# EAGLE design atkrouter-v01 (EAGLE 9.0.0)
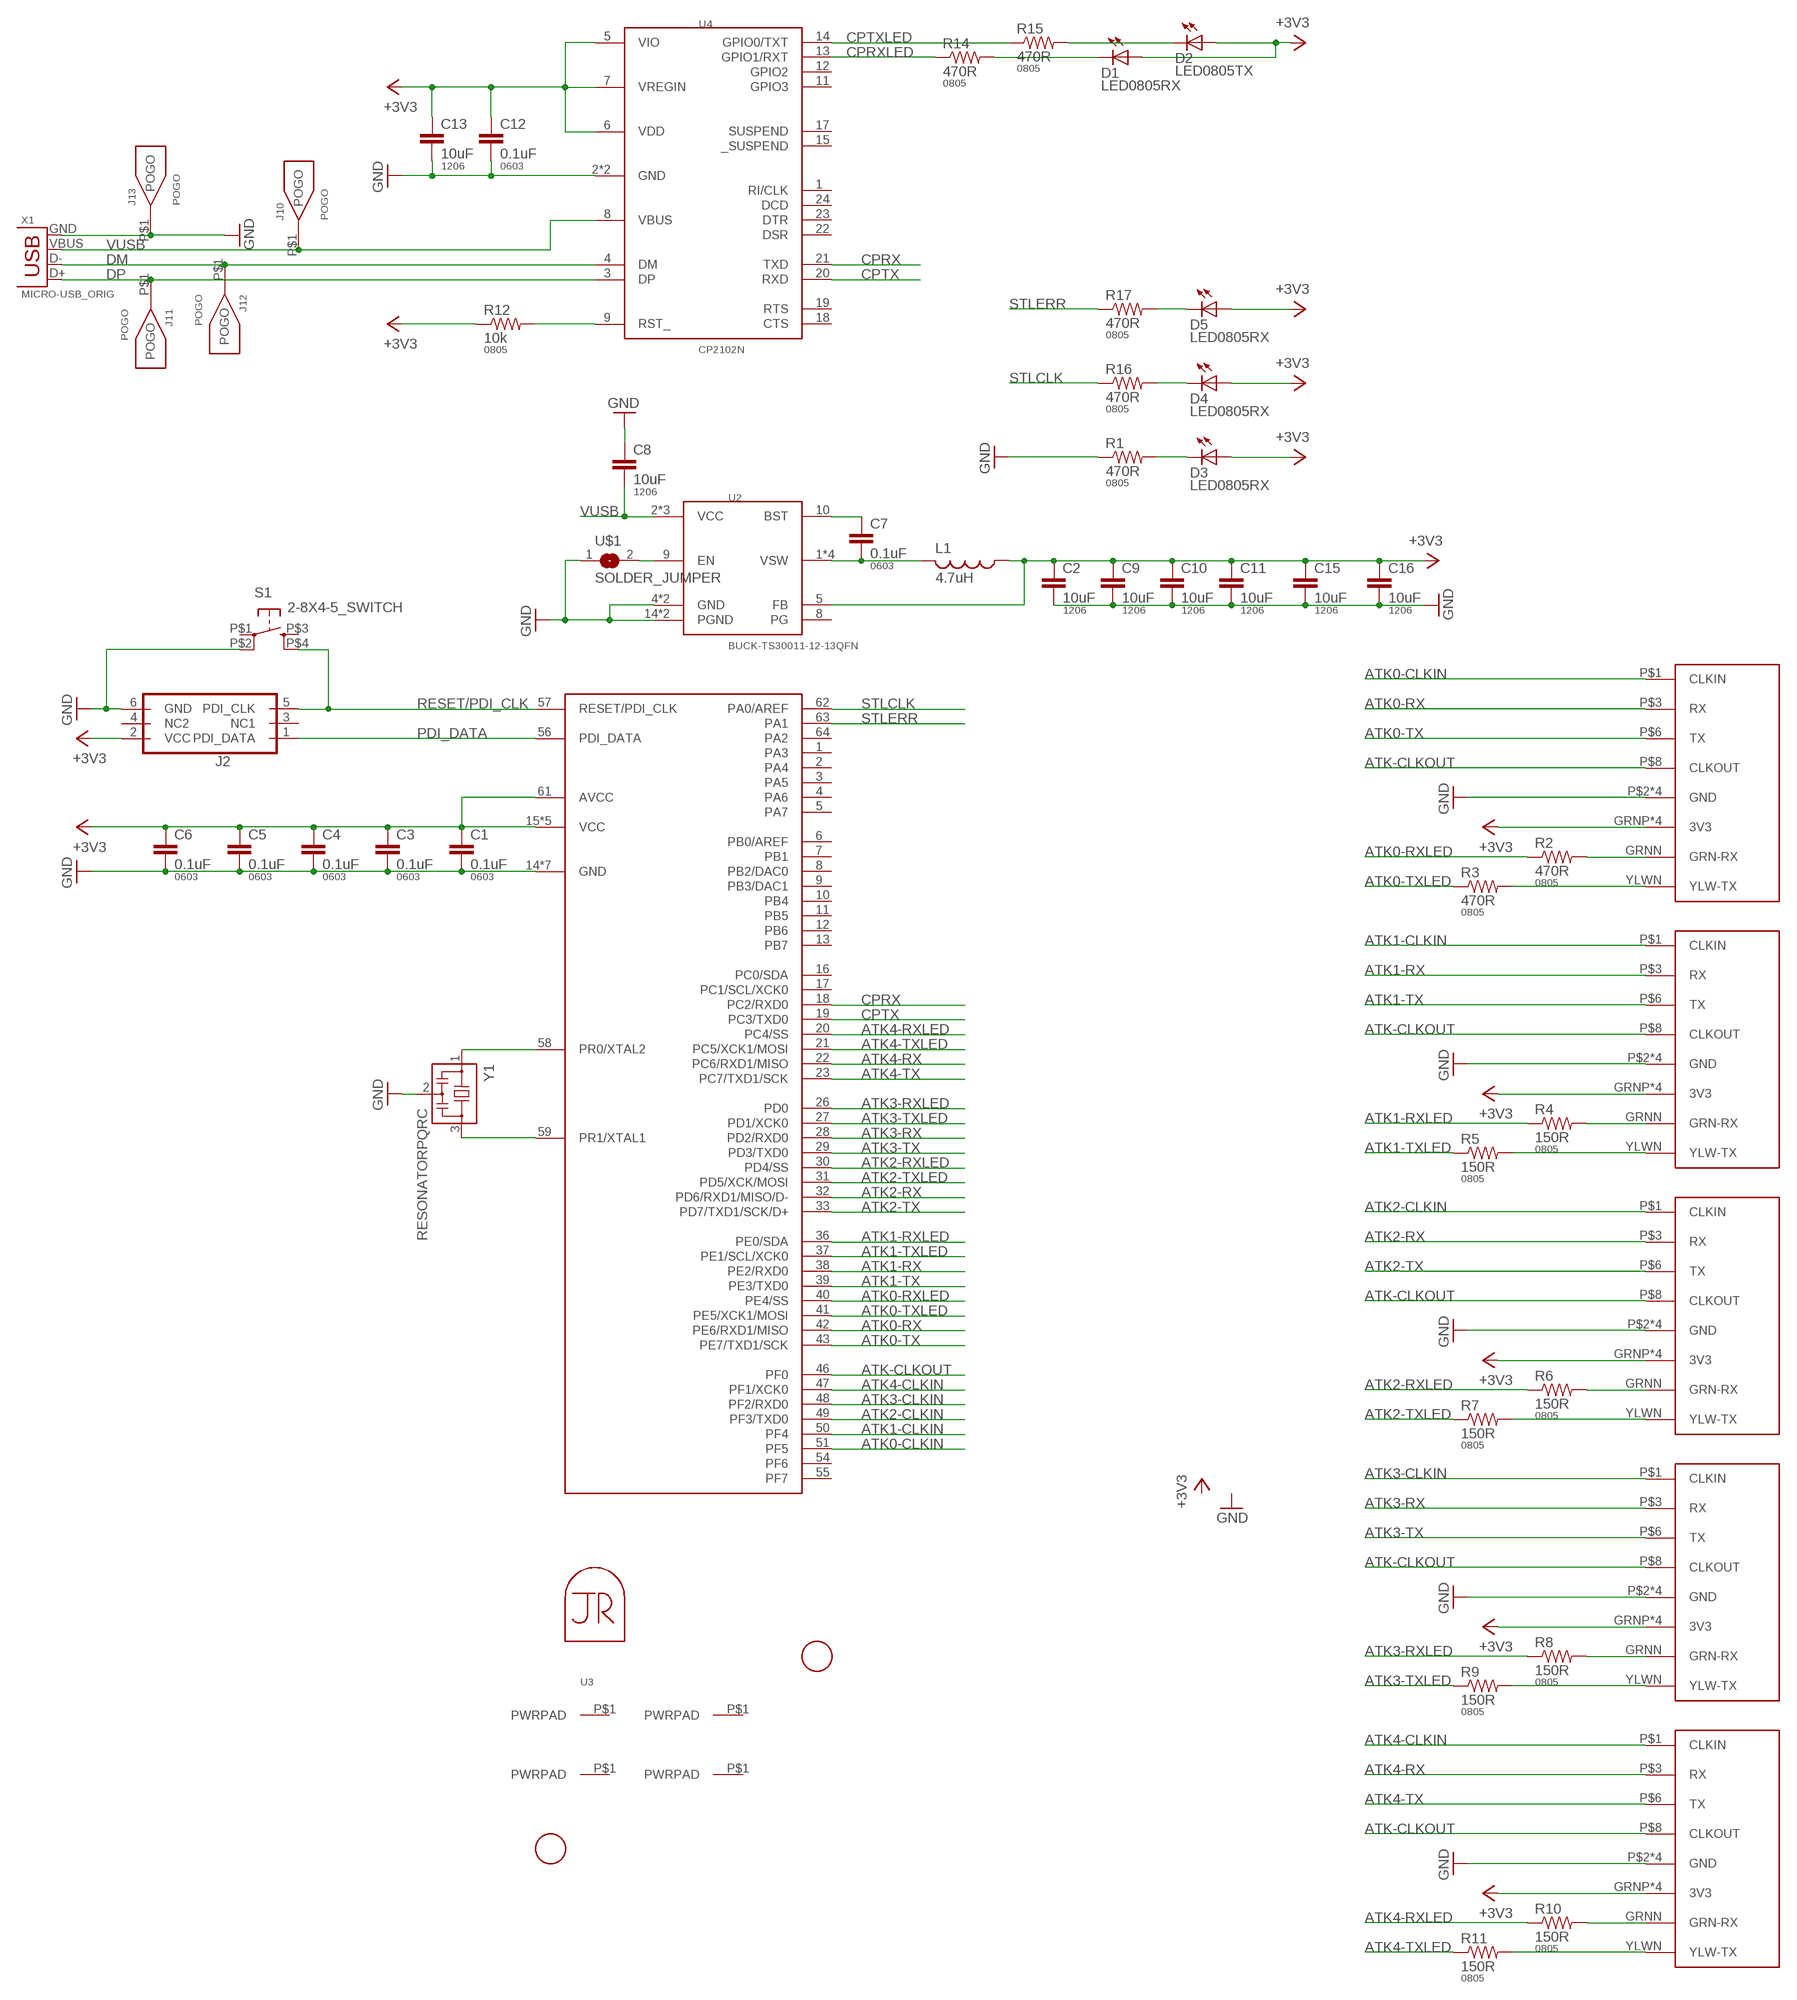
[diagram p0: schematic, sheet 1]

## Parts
C1  0.1uF  CAP0603-CAP  [0603-CAP]
C2  10uF  CAP1206  [1206]
C3  0.1uF  CAP0603-CAP  [0603-CAP]
C4  0.1uF  CAP0603-CAP  [0603-CAP]
C5  0.1uF  CAP0603-CAP  [0603-CAP]
C6  0.1uF  CAP0603-CAP  [0603-CAP]
C7  0.1uF  CAP0603-CAP  [0603-CAP]
C8  10uF  CAP1206  [1206]
C9  10uF  CAP1206  [1206]
C10  10uF  CAP1206  [1206]
C11  10uF  CAP1206  [1206]
C12  0.1uF  CAP0603-CAP  [0603-CAP]
C13  10uF  CAP1206  [1206]
C15  10uF  CAP1206  [1206]
C16  10uF  CAP1206  [1206]
D1  LED0805RX  LED0805  [LED0805]
D2  LED0805TX  LED0805  [LED0805]
D3  LED0805RX  LED0805  [LED0805]
D4  LED0805RX  LED0805  [LED0805]
D5  LED0805RX  LED0805  [LED0805]
J1  PWRPADM2.5  [PWRPAD_2-65MM]
J2  PDIFEMALE_SMD  [PDI_2X3_SMD]
J3  ATK-PHY  [RJ45-LED-RJE7318800XXX]
J4  ATK-PHY  [RJ45-LED-RJE7318800XXX]
J5  ATK-PHY  [RJ45-LED-RJE7318800XXX]
J6  ATK-PHY  [RJ45-LED-RJE7318800XXX]
J7  ATK-PHY  [RJ45-LED-RJE7318800XXX]
J8  PWRPADM2.5  [PWRPAD_2-65MM]
J9  PWRPADM2.5  [PWRPAD_2-65MM]
J10  POGO  [POGO]
J11  POGO  [POGO]
J12  POGO  [POGO]
J13  POGO  [POGO]
J14  PWRPADM2.5  [PWRPAD_2-65MM]
L1  4.7uH  INDUCTOR  [NRS5020T4R7MMGJ]
MP1  JRTOMBSTONE  [JRTOMBSTONE]
R1  470R  RESISTOR0805-RES  [0805]
R2  470R  RESISTOR0805-RES  [0805]
R3  470R  RESISTOR0805-RES  [0805]
R4  150R  RESISTOR0805-RES  [0805]
R5  150R  RESISTOR0805-RES  [0805]
R6  150R  RESISTOR0805-RES  [0805]
R7  150R  RESISTOR0805-RES  [0805]
R8  150R  RESISTOR0805-RES  [0805]
R9  150R  RESISTOR0805-RES  [0805]
R10  150R  RESISTOR0805-RES  [0805]
R11  150R  RESISTOR0805-RES  [0805]
R12  10k  RESISTOR0805-RES  [0805]
R14  470R  RESISTOR0805-RES  [0805]
R15  470R  RESISTOR0805-RES  [0805]
R16  470R  RESISTOR0805-RES  [0805]
R17  470R  RESISTOR0805-RES  [0805]
S1  2-8X4-5_SWITCH  [TACT-SWITCH-KMR6]
U1  ATXMEGA_A3UQFN  [QFN-64-9X9MM]
U2  BUCK-TS30011-12-13QFN  [QFN16-3X3-TI-RTE]
U3  RASPBERRYPI-3BPLUS  [RASPBERRYPI-3BPLUS]
U4  CP2102N  [QFN-24_ALT2]
U$1  SOLDER_JUMPER  [SJFAB]
U$3  FIDUCIAL  [FIDUCIAL_1MM]
U$4  FIDUCIAL  [FIDUCIAL_1MM]
X1  MICRO-USB_ORIG  [DX4R005HJ5]
Y1  RESONATORPQRC  [RES_PRQC]

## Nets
+3V3: C1.1 C2.1 C3.1 C4.1 C5.1 C6.1 C9.1 C10.1 C11.1 C12.1 C13.1 C15.1 C16.1 D1.1(A) D2.1(A) D3.1(A) D4.1(A) D5.1(A) J2.2(VCC) J3.GRNP(3V3) J3.P$4(3V3) J3.P$5(3V3) J3.YLWP(3V3) J4.GRNP(3V3) J4.P$4(3V3) J4.P$5(3V3) J4.YLWP(3V3) J5.GRNP(3V3) J5.P$4(3V3) J5.P$5(3V3) J5.YLWP(3V3) J6.GRNP(3V3) J6.P$4(3V3) J6.P$5(3V3) J6.YLWP(3V3) J7.GRNP(3V3) J7.P$4(3V3) J7.P$5(3V3) J7.YLWP(3V3) L1.1 R12.1 U1.15(VCC) U1.25(VCC) U1.35(VCC) U1.45(VCC) U1.53(VCC) U1.61(AVCC) U2.5(FB) U4.5(VIO) U4.6(VDD) U4.7(VREGIN)
ATK0-CLKIN: J3.P$1(CLKIN) U1.51(PF5)
ATK0-RX: J3.P$3(RX) U1.42(PE6/RXD1/MISO)
ATK0-RXLED: R2.1 U1.40(PE4/SS)
ATK0-TX: J3.P$6(TX) U1.43(PE7/TXD1/SCK)
ATK0-TXLED: R3.1 U1.41(PE5/XCK1/MOSI)
ATK1-CLKIN: J4.P$1(CLKIN) U1.50(PF4)
ATK1-RX: J4.P$3(RX) U1.38(PE2/RXD0)
ATK1-RXLED: R4.1 U1.36(PE0/SDA)
ATK1-TX: J4.P$6(TX) U1.39(PE3/TXD0)
ATK1-TXLED: R5.1 U1.37(PE1/SCL/XCK0)
ATK2-CLKIN: J5.P$1(CLKIN) U1.49(PF3/TXD0)
ATK2-RX: J5.P$3(RX) U1.32(PD6/RXD1/MISO/D-)
ATK2-RXLED: R6.1 U1.30(PD4/SS)
ATK2-TX: J5.P$6(TX) U1.33(PD7/TXD1/SCK/D+)
ATK2-TXLED: R7.1 U1.31(PD5/XCK/MOSI)
ATK3-CLKIN: J6.P$1(CLKIN) U1.48(PF2/RXD0)
ATK3-RX: J6.P$3(RX) U1.28(PD2/RXD0)
ATK3-RXLED: R8.1 U1.26(PD0)
ATK3-TX: J6.P$6(TX) U1.29(PD3/TXD0)
ATK3-TXLED: R9.1 U1.27(PD1/XCK0)
ATK4-CLKIN: J7.P$1(CLKIN) U1.47(PF1/XCK0)
ATK4-RX: J7.P$3(RX) U1.22(PC6/RXD1/MISO)
ATK4-RXLED: R10.1 U1.20(PC4/SS)
ATK4-TX: J7.P$6(TX) U1.23(PC7/TXD1/SCK)
ATK4-TXLED: R11.1 U1.21(PC5/XCK1/MOSI)
ATK-CLKOUT: J3.P$8(CLKOUT) J4.P$8(CLKOUT) J5.P$8(CLKOUT) J6.P$8(CLKOUT) J7.P$8(CLKOUT) U1.46(PF0)
CPRX: U1.18(PC2/RXD0) U4.21(TXD)
CPRXLED: R14.1 U4.13(GPIO1/RXT)
CPTX: U1.19(PC3/TXD0) U4.20(RXD)
CPTXLED: R15.1 U4.14(GPIO0/TXT)
DM: J12.P$1(POGO) U4.4(DM) X1.D-
DP: J11.P$1(POGO) U4.3(DP) X1.D+
GND: C1.2 C2.2 C3.2 C4.2 C5.2 C6.2 C8.1 C9.2 C10.2 C11.2 C12.2 C13.2 C15.2 C16.2 J2.6(GND) J3.P$2(GND) J3.P$7(GND) J3.SHDL1(GND) J3.SHDL2(GND) J4.P$2(GND) J4.P$7(GND) J4.SHDL1(GND) J4.SHDL2(GND) J5.P$2(GND) J5.P$7(GND) J5.SHDL1(GND) J5.SHDL2(GND) J6.P$2(GND) J6.P$7(GND) J6.SHDL1(GND) J6.SHDL2(GND) J7.P$2(GND) J7.P$7(GND) J7.SHDL1(GND) J7.SHDL2(GND) J13.P$1(POGO) R1.1 S1.P$2(P1) U1.14(GND) U1.24(GND) U1.34(GND) U1.44(GND) U1.52(GND) U1.60(GND) U1.P$1(GND) U2.4(GND) U2.14(PGND) U2.15(PGND) U2.TH(GND) U4.2(GND) U4.EP(GND) U$1.1 X1.GND Y1.2
N$1: J3.GRNN(GRN-RX) R2.2
N$2: J3.YLWN(YLW-TX) R3.2
N$3: J4.GRNN(GRN-RX) R4.2
N$4: J4.YLWN(YLW-TX) R5.2
N$5: J5.GRNN(GRN-RX) R6.2
N$6: J5.YLWN(YLW-TX) R7.2
N$7: J6.GRNN(GRN-RX) R8.2
N$8: J6.YLWN(YLW-TX) R9.2
N$9: J7.GRNN(GRN-RX) R10.2
N$10: J7.YLWN(YLW-TX) R11.2
N$13: U1.58(PR0/XTAL2) Y1.1
N$14: U1.59(PR1/XTAL1) Y1.3
N$15: D3.2(C) R1.2
N$17: D4.2(C) R16.2
N$19: R12.2 U4.9(RST_)
N$20: C7.1 U2.10(BST)
N$21: D5.2(C) R17.2
N$34: U2.9(EN) U$1.2
N$37: D1.2(C) R14.2
N$38: D2.2(C) R15.2
PDI_DATA: J2.1(PDI_DATA) U1.56(PDI_DATA)
RESET/PDI_CLK: J2.5(PDI_CLK) S1.P$4(S1) U1.57(RESET/PDI_CLK)
STLCLK: R16.1 U1.62(PA0/AREF)
STLERR: R17.1 U1.63(PA1)
VSW: C7.2 L1.2 U2.1(VSW) U2.12(VSW) U2.13(VSW) U2.16(VSW)
VUSB: C8.2 J10.P$1(POGO) U2.2(VCC) U2.3(VCC) U2.11(VCC) U4.8(VBUS) X1.VBUS
Unconnected: J1.P$1(PWRPAD) J2.3(NC1) J2.4(NC2) J8.P$1(PWRPAD) J9.P$1(PWRPAD) J14.P$1(PWRPAD) S1.P$1(P) S1.P$3(S) U1.1(PA3) U1.2(PA4) U1.3(PA5) U1.4(PA6) U1.5(PA7) U1.6(PB0/AREF) U1.7(PB1) U1.8(PB2/DAC0) U1.9(PB3/DAC1) U1.10(PB4) U1.11(PB5) U1.12(PB6) U1.13(PB7) U1.16(PC0/SDA) U1.17(PC1/SCL/XCK0) U1.54(PF6) U1.55(PF7) U1.64(PA2) U2.8(PG) U4.1(RI/CLK) U4.11(GPIO3) U4.12(GPIO2) U4.15(_SUSPEND) U4.17(SUSPEND) U4.18(CTS) U4.19(RTS) U4.22(DSR) U4.23(DTR) U4.24(DCD)

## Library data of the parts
C1 C3-C7 C12 = passives:CAP: Capacitor; PACKAGE: 0603
C2 C8-C11 C13 C15 C16 = passives:CAP: Capacitor; PACKAGE: 1206
D1-D5 = lights:LED: LED
J1 J8 J9 J14 = power:PWRPAD
J2 = microcontrollers:PDI: Multi connection point. Often used as Generic Header-pin footprint for 0.1 inch spaced/style header connections You can populate with any combo of single row headers, but if you'd like an exact match, check these: Header - 2x3 (Male, 0.1") (PRT-12807) Header - 2x3 (Female, 0.1") (PRT-13010) 2x3 Pin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; PROD_ID: CONN-11290
J3-J7 = connector:ATK-PHY
J10-J13 = connector:POGO
L1 = power:INDUCTOR
MP1 = connector:JRTOMBSTONE
R1-R12 R14-R17 = passives:RESISTOR: Resistor; PACKAGE: 0805
S1 = passives:2-8X4-5_SWITCH
U1 = microcontrollers:ATXMEGA_A3U
U2 = power:BUCK-TS30011-12-13
U3 = connector:RASPBERRYPI-3BPLUS
U4 = microcontrollers:CP2102N
U$1 = connector:SOLDER_JUMPER
U$3 U$4 = connector:FIDUCIAL: For use by pick and place machines to calibrate the vision/machine, 1mm
X1 = connector:MICRO-USB: SMD micro USB connector as found in the fablab inventory. Three footprint variants included: original, as described by manufacturer's datasheet for milling with the 1/100" bit for milling with the 1/64" bit Made by Zaerc.
Y1 = passives:RESONATOR

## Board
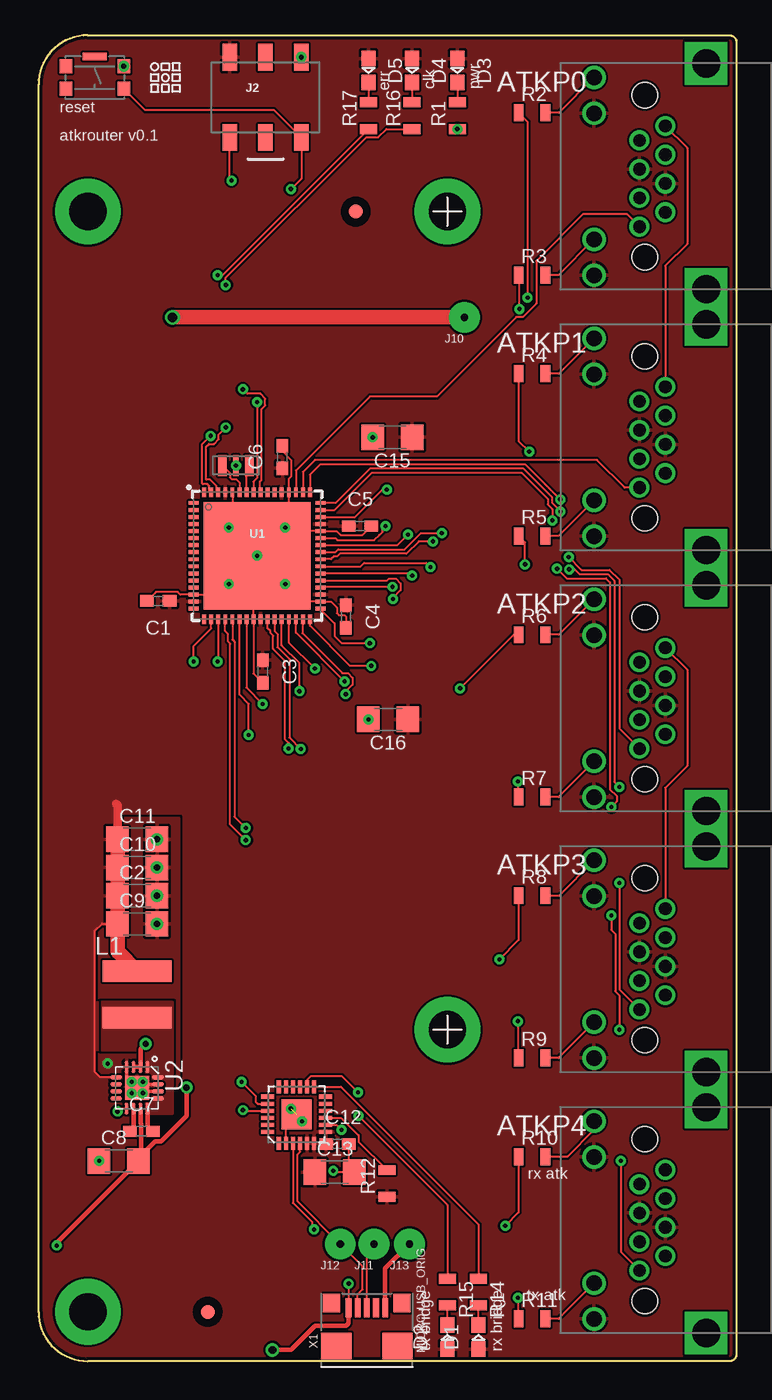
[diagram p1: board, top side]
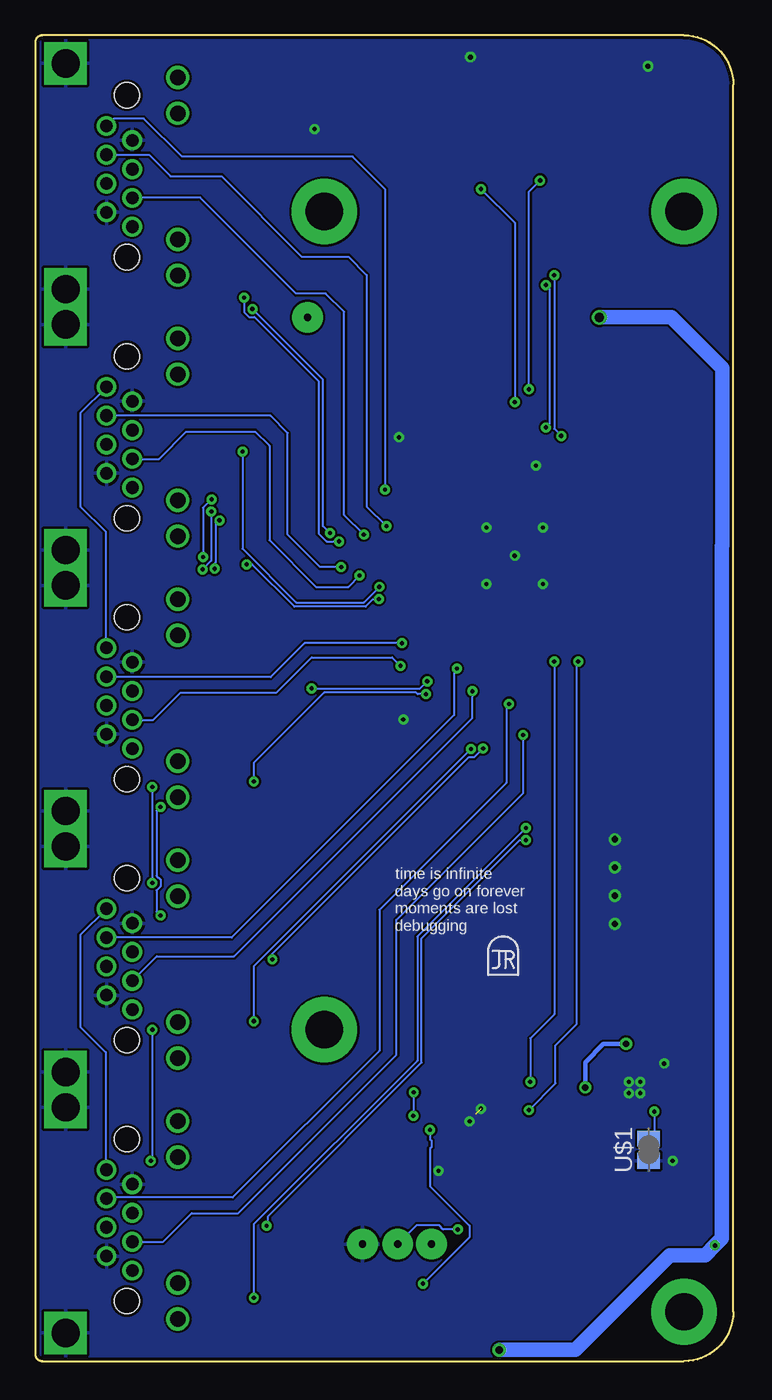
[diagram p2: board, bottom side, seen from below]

Size 49.5 x 94 mm. Coordinates in mm from the lower left corner, seen from the top.
Outline: 49,0 3.5,0 arc-90 0,3.5 0,90.5 arc-90 3.5,94 49,94 arc-90 49.5,93.5 49.5,0.5 arc-90 49,0
Copper layers (1*16): Top 0.035mm / dielectric 1.5mm / Bottom 0.035mm
Design rules "default *": minimum track width 6mil, minimum drill 0.3mm, track to track 6mil, track to pad 6mil, pad to pad 6mil, via to via 6mil, smd to smd 6mil, copper to edge 8mil, drill to drill 6mil, minimum pad ring 10mil, minimum via ring 8mil, stop-mask expansion 4mil, vias tented up to drill 25mil, thermal gap 8mil

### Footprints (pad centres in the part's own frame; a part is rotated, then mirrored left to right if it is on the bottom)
0603-CAP = smd 0.96 x 0.8: 1 -0.8,0; 2 0.8,0
1206 = smd 1.6 x 1.8: 1 -1.4,0; 2 1.4,0
LED0805 = smd 1.1 x 1: 1 -0.85,0; 2 0.85,0
PWRPAD_2-65MM = drill 2.65 pad 4.65: P$1 0,0
PDI_2X3_SMD = smd 1.02 x 1.9: 1 -2.54,-2.85; 2 -2.54,2.85; 3 0,-2.85; 4 0,2.85; 5 2.54,-2.85; 6 2.54,2.85
RJ45-LED-RJE7318800XXX = drill 1.1: GRNN 7.01,3.6; GRNP 4.47,3.6; YLWN -4.47,3.6; YLWP -7.01,3.6 | drill 0.9: P$1 -3.57,0.38; P$2 -2.55,-1.45; P$3 -1.53,0.38; P$4 -0.51,-1.45; P$5 0.51,0.38; P$6 1.53,-1.45; P$7 2.55,0.38; P$8 3.57,-1.45 | drill 2 square: SHDL1 -8,-4.35; SHDL2 8,-4.35 | hole 1.8: -5.74,0; 5.74,0
POGO = drill 0.51 pad 2.184: P$1 0,0
NRS5020T4R7MMGJ = smd 4.9 x 1.5: 1 0,1.65; 2 0,-1.65
0805 = smd 0.7 x 1.2: 1 -0.95,0; 2 0.95,0
TACT-SWITCH-KMR6 = smd 0.9 x 1: P$1 -2.05,0.8; P$2 2.05,0.8; P$3 -2.05,-0.8; P$4 2.05,-0.8 | smd 1.7 x 0.55: P$5 0,1.5
QFN-64-9X9MM = smd 0.7 x 0.275: 1 -4.5,3.75; 2 -4.5,3.25; 3 -4.5,2.75; 4 -4.5,2.25; 5 -4.5,1.75; 6 -4.5,1.25; 7 -4.5,0.75; 8 -4.5,0.25; 9 -4.5,-0.25; 10 -4.5,-0.75; 11 -4.5,-1.25; 12 -4.5,-1.75; 13 -4.5,-2.25; 14 -4.5,-2.75; 15 -4.5,-3.25; 16 -4.5,-3.75; 33 4.5,-3.75; 34 4.5,-3.25; 35 4.5,-2.75; 36 4.5,-2.25; 37 4.5,-1.75; 38 4.5,-1.25; 39 4.5,-0.75; 40 4.5,-0.25; 41 4.5,0.25; 42 4.5,0.75; 43 4.5,1.25; 44 4.5,1.75; 45 4.5,2.25; 46 4.5,2.75; 47 4.5,3.25; 48 4.5,3.75 | smd 0.275 x 0.7: 17 -3.75,-4.5; 18 -3.25,-4.5; 19 -2.75,-4.5; 20 -2.25,-4.5; 21 -1.75,-4.5; 22 -1.25,-4.5; 23 -0.75,-4.5; 24 -0.25,-4.5; 25 0.25,-4.5; 26 0.75,-4.5; 27 1.25,-4.5; 28 1.75,-4.5; 29 2.25,-4.5; 30 2.75,-4.5; 31 3.25,-4.5; 32 3.75,-4.5; 49 3.75,4.5; 50 3.25,4.5; 51 2.75,4.5; 52 2.25,4.5; 53 1.75,4.5; 54 1.25,4.5; 55 0.75,4.5; 56 0.25,4.5; 57 -0.25,4.5; 58 -0.75,4.5; 59 -1.25,4.5; 60 -1.75,4.5; 61 -2.25,4.5; 62 -2.75,4.5; 63 -3.25,4.5; 64 -3.75,4.5 | smd 7.6 x 7.6: P$1 0,0
QFN16-3X3-TI-RTE = smd 0.85 x 0.3: 1 -1.475,0.75; 2 -1.475,0.25; 3 -1.475,-0.25; 4 -1.475,-0.75; 9 1.475,-0.75; 10 1.475,-0.25; 11 1.475,0.25; 12 1.475,0.75 | smd 0.3 x 0.85: 5 -0.75,-1.475; 6 -0.25,-1.475; 7 0.25,-1.475; 8 0.75,-1.475; 13 0.75,1.475; 14 0.25,1.475; 15 -0.25,1.475; 16 -0.75,1.475 | smd 1.7 x 1.7: TH 0,0
QFN-24_ALT2 = smd 0.9 x 0.3: 1 -2.05,1.25; 2 -2.05,0.75; 3 -2.05,0.25; 4 -2.05,-0.25; 5 -2.05,-0.75; 6 -2.05,-1.25; 13 1.95,-1.25; 14 1.95,-0.75; 15 1.95,-0.25; 16 1.95,0.25; 17 1.95,0.75; 18 1.95,1.25 | smd 0.3 x 0.9: 7 -1.25,-2.05; 8 -0.75,-2.05; 9 -0.25,-2.05; 10 0.25,-2.05; 11 0.75,-2.05; 12 1.25,-2.05; 19 1.25,2.05; 20 0.75,2.05; 21 0.25,2.05; 22 -0.25,2.05; 23 -0.75,2.05; 24 -1.25,2.05 | smd 2.1 x 2.1: EP 0,0
SJFAB = smd 1.118 x 1.6: 1 -0.787,0; 2 0.787,0
FIDUCIAL_1MM = smd 1 x 1: 1 0,0
DX4R005HJ5 = smd 0.4 x 1.35: D+ 0,1.6; D- -0.65,1.6; GND 1.3,1.6; ID 0.65,1.6; VBUS -1.3,1.6 | smd 1.2 x 1.3: GND@1 -2.5,1.95; GND@2 2.5,1.95 | smd 2.15 x 1.9: GND@3 -2.175,-1.1; GND@4 2.175,-1.1
RES_PRQC = smd 0.6 x 1.5: 1 -0.95,0; 3 0.95,0 | smd 0.4 x 1.5: 2 0,0

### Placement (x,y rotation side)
C1  8.5,53.9 180 top
C2  7,33 0 top
C3  15.9,48.9 270 top
C4  21.8,52.8 270 top
C5  22.8,59.2 0 top
C6  17.3,64.1 90 top
C7  7.3,16.3 0 top
C8  5.7,14.2 0 top
C9  7,31 0 top
C10  7,35 0 top
C11  7,37 0 top
C12  21.2,15.4 0 top
C13  21,13.4 0 top
C15  25.1,65.5 180 top
C16  24.8,45.5 180 top
D1  31.2,1.7 90 top
D2  29,1.7 90 top
D3  29.7,91.5 270 top
D4  26.5,91.5 270 top
D5  23.4,91.5 270 top
J1  29,23.5 0 top
J2  16.1,89.6 0 top
J3  43,84 90 top
J4  43,65.5 90 top
J5  43,47 90 top
J6  43,28.5 90 top
J7  43,10 90 top
J8  3.5,3.5 0 top
J9  29,81.5 0 top
J10  30.2,74 0 top
J11  23.8,8.3 0 top
J12  21.4,8.3 0 top
J13  26.3,8.3 0 top
J14  3.5,81.5 0 top
L1  7,26 0 top
MP1  16.27,28.38 0 bottom
R1  29.7,88.3 90 top
R2  35,88.5 0 top
R3  35,77 0 top
R4  35,70 0 top
R5  35,58.5 0 top
R6  35,51.5 0 top
R7  35,40 0 top
R8  35,33 0 top
R9  35,21.5 0 top
R10  35,14.5 0 top
R11  35,3 0 top
R12  24.7,12.6 90 top
R14  31.2,4.9 270 top
R15  29,4.9 270 top
R16  26.5,88.3 90 top
R17  23.4,88.3 90 top
S1  4,91 0 top
U1  15.5,57.1 0 top
U2  6.99,19.38 270 top
U3  not placed on the board
U4  18.3,17.5 90 top
U$1  6,15 90 bottom
U$2  CBA-LOGO  [CBA-SILK-LOGO]  9,91 0 top
U$3  12,3.5 0 top
U$4  22.5,81.5 0 top
X1  23.29,2.18 0 top
Y1  14,63.5 180 top

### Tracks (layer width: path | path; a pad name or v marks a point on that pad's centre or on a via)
+3V3
  Top 0.152: U2.5 4.37,20.13 4,20.5 4,30.5 4.5,31 C9.1
  Top 0.61: C11.1 5.6,39.4 5.5,39.5
  Top 1.016: L1.1 5.6,29.05 C9.1 C2.1 C10.1 C11.1
  pour Top (rank 6): -1,114 51,114 51,-1.5 -1,-1.5
ATK0-CLKIN
  Top 0.152: J3.P$1 41.75,81.3 38.6,81.3 35.3,78 35.3,74.98 34.34,74.02 33.89,74.02 28.27,68.4 23.5,68.4 18.25,63.15 U1.51
ATK0-RX  (via drill 0.3)
  Top 0.152: U1.42 25.45,57.85 v26.2,58.6
  Bottom 0.152: v26.2,58.6 27.6,60 27.6,74.4 28.9,75.7 31,75.7 37.8,82.5 42.59,82.5 J3.P$3
ATK0-RXLED  (via drill 0.3)
  Top 0.152: R2.1 34.68,87.87 v34.68,75.4 | v27.97,58.12 26.97,58.12 26.09,57.24 21.37,57.24 21.18,57.05 20.95,57.05 20.75,56.85 U1.40
  Bottom 0.152: v34.68,75.4 34.68,74.36 34.34,74.02 33.95,74.02 29.41,69.47 29.41,58.68 28.84,58.12 v27.97,58.12
ATK0-TX  (via drill 0.3)
  Top 0.152: U1.43 21.05,58.35 21.2,58.2 23.8,58.2 24.17,58.57 24.18,58.57 24.4,58.8 24.4,59 v24.6,59.2
  Bottom 0.152: J3.P$6 41.43,85.53 39.9,84 36.3,84 30.6,78.3 27.3,78.3 26,77 26,60.6 v24.6,59.2
ATK0-TXLED  (via drill 0.3)
  Top 0.152: U1.41 21.05,57.35 21.25,57.55 25.97,57.55 27.12,58.7 v28.6,58.7 | v34.1,74.6 34.1,76.95 R3.1
  Bottom 0.152: v28.6,58.7 29.1,59.2 29.1,69.6 v34.1,74.6
ATK1-CLKIN
  Top 0.152: J4.P$1 41.57,61.93 39.6,63.9 19.6,63.9 18.75,63.05 U1.50
ATK1-RX  (via drill 0.3)
  Top 0.152: v26.5,55.7 26.35,55.85 U1.38
  Bottom 0.152: J4.P$3 40.73,63.97 38.8,65.9 33.9,65.9 32.9,64.9 32.9,58.2 29.6,54.9 27.3,54.9 v26.5,55.7
ATK1-RXLED  (via drill 0.3)
  Top 0.152: R4.1 34.05,65.23 v34.8,64.48 | v25.1,54.9 20.05,54.9 U1.36
  Bottom 0.152: v34.8,64.48 34.8,57.6 31,53.8 26.2,53.8 v25.1,54.9
ATK1-TX  (via drill 0.3)
  Top 0.152: U1.39 22.85,56.35 23.1,56.6 27.5,56.6 v27.8,56.3
  Bottom 0.152: v27.8,56.3 29.3,56.3 31.6,58.6 31.6,65.8 32.83,67.03 J4.P$6
ATK1-TXLED  (via drill 0.3)
  Top 0.152: v25.14,54.04 25.14,54.12 25.68,54.66 25.68,55.14 25.34,55.48 24.86,55.48 24.73,55.35 U1.37 | v34.51,56.49 34.51,58.04 R5.1
  Bottom 0.152: v25.14,54.04 25.18,54 25.57,54 26.07,53.49 31.13,53.49 34.12,56.49 v34.51,56.49
ATK2-CLKIN  (via drill 0.3)
  Top 0.152: v37,61.1 34.51,63.59 20,63.59 19.25,62.85 U1.49 | v37.6,57 38.5,56.1 40.5,56.1 41.2,55.4 41.2,44.85 J5.P$1
  Bottom 0.152: v37,61.1 37.6,60.5 v37.6,57
ATK2-RX  (via drill 0.3)
  Top 0.152: v23.6,49.3 22.1,49.3 19.25,52.15 U1.32
  Bottom 0.152: J5.P$3 41.13,45.47 39.2,47.4 32.4,47.4 29.9,49.9 24.2,49.9 v23.6,49.3
ATK2-RXLED  (via drill 0.3)
  Top 0.152: R6.1 33.7,51.5 v29.9,47.7 | v21.7,48.2 18.25,51.65 U1.30
  Bottom 0.152: v29.9,47.7 22.2,47.7 v21.7,48.2
ATK2-TX  (via drill 0.3)
  Top 0.152: U1.33 20,53.3 21,52.3 21,51.4 21.5,50.9 v23.5,50.9
  Bottom 0.152: v23.5,50.9 30.4,50.9 32.8,48.5 44.42,48.5 J5.P$6
ATK2-TXLED  (via drill 0.3)
  Top 0.152: U1.31 18.72,52.57 18.72,51.62 21.55,48.78 21.94,48.78 22.28,48.44 22.28,47.96 21.79,47.47 v21.79,47.29 | v34,41.1 34,40.05 R7.1
  Bottom 0.152: v21.79,47.29 22.39,47.29 22.5,47.4 29,47.4 34,42.4 v34,41.1
ATK3-CLKIN  (via drill 0.3)
  Top 0.152: v37.02,60.24 37.02,60.26 36.42,60.86 36.42,61.25 34.38,63.29 23.52,63.29 21.08,60.85 U1.48 | v37.64,56.14 38.03,56.14 38.37,55.8 40.37,55.8 40.83,55.33 40.83,41.07 v41.2,40.7 | v41.2,33.9 41.2,26.35 J6.P$1
  Bottom 0.152: v37.02,60.24 37.02,56.76 v37.64,56.14 | v41.2,40.7 v41.2,33.9
ATK3-RX  (via drill 0.3)
  Top 0.152: v18.5,47.5 18.5,49.5 17.25,50.75 U1.28
  Bottom 0.152: J6.P$3 40.89,28.7 35.4,28.7 18.5,45.6 v18.5,47.5
ATK3-RXLED  (via drill 0.3)
  Top 0.152: R8.1 34.05,29.85 v32.69,28.49 | v17.74,43.44 17.74,43.83 17.5,44.07 17.5,49.64 16.64,50.5 16.64,51.43 16.45,51.62 16.45,51.76 16.25,51.95 U1.26
  Bottom 0.152: v32.69,28.49 32.69,28.88 18.75,42.82 18.36,42.82 v17.74,43.44
ATK3-TX  (via drill 0.3)
  Top 0.152: U1.29 17.75,50.95 v19.6,49.1
  Bottom 0.152: v19.6,49.1 19.8,48.9 19.8,45.8 35.57,30.03 J6.P$6
ATK3-TXLED  (via drill 0.3)
  Top 0.152: U1.27 16.75,51.75 16.95,51.55 16.95,50.62 17.8,49.77 17.8,44.2 v18.6,43.4 | v34,24.1 34,21.55 R9.1
  Bottom 0.152: v18.6,43.4 34,28 v34,24.1
ATK4-CLKIN  (via drill 0.3)
  Top 0.152: v36.44,59.61 36.44,60.41 36.11,60.73 36.11,61.12 34.25,62.99 23.65,62.99 21.01,60.35 U1.47 | v36.78,56.18 37.46,55.49 40.25,55.49 40.53,55.21 40.53,40.55 41,40.08 41,39.68 v40.62,39.3 | v40.62,31.6 40.62,30.58 40.9,30.3 40.9,26.22 41.2,25.92 v41.2,23.5 | v41.3,14.2 41.3,7.75 J7.P$1
  Bottom 0.152: v36.44,59.61 36.59,59.61 36.71,59.49 36.71,56.63 36.78,56.57 v36.78,56.18 | v40.62,39.3 40.9,39.02 40.9,34.42 40.62,34.14 40.62,33.66 40.9,33.38 40.9,31.88 v40.62,31.6 | v41.2,23.5 41.2,14.3 v41.3,14.2
ATK4-RX  (via drill 0.3)
  Top 0.152: U1.22 14.25,47.25 14.9,46.6 v14.9,44.4
  Bottom 0.152: J7.P$3 40.43,8.47 38.4,10.5 35.1,10.5 23.9,21.7 23.9,31.3 14.9,40.3 v14.9,44.4
ATK4-RXLED  (via drill 0.3)
  Top 0.152: R10.1 34.05,10.55 v33.1,9.6 | v14.7,36.94 13.6,38.05 13.6,50.87 13.45,51.02 13.45,51.55 13.25,51.75 U1.20
  Bottom 0.152: v33.1,9.6 33,9.7 33,10.27 22.09,21.17 22.09,29.97 15.13,36.94 v14.7,36.94
ATK4-TX  (via drill 0.3)
  Top 0.152: U1.23 14.75,47.75 v15.9,46.6
  Bottom 0.152: v15.9,46.6 16.1,46.4 16.1,41 25.1,32 25.1,22 35.5,11.6 44.38,11.6 J7.P$6
ATK4-TXLED  (via drill 0.3)
  Top 0.152: U1.21 13.75,51.15 13.9,51 13.9,38.6 v14.7,37.8 | v34,4.5 34,3.05 R11.1
  Bottom 0.152: v14.7,37.8 22.4,30.1 22.4,21.3 34,9.7 v34,4.5
ATK-CLKOUT  (via drill 0.3)
  Top 0.152: J3.P$8 46,86.02 46,79.2 44.45,77.65 J4.P$8 | J5.P$8 46,49.02 46,42.2 44.45,40.65 J6.P$8 | U1.46 22.45,59.85 24.4,61.8 v24.7,61.8
  Bottom 0.152: J3.P$8 43.92,88.1 41.8,88.1 39.1,85.4 27,85.4 24.7,83.1 v24.7,61.8 | J4.P$8 46.3,67.22 46.3,60.6 44.5,58.8 44.5,50.62 J5.P$8 | J6.P$8 46.3,30.22 46.3,23.7 44.5,21.9 44.5,13.62 J7.P$8
CPRX  (via drill 0.3)
  Top 0.152: v11,49.6 11,50.7 12.25,51.95 U1.18 | v14.5,17.8 14.55,17.75 U4.21
  Bottom 0.152: v14.5,17.8 12.6,19.7 12.6,22.4 11.1,23.9 11.1,49.5 v11,49.6
CPRXLED
  Top 0.152: R14.1 31.2,9.7 21.45,19.45 U4.13
CPTX  (via drill 0.3)
  Top 0.152: U1.19 12.75,49.65 v12.7,49.6 | v14.4,19.8 15.4,18.8 15.4,18.4 15.55,18.25 U4.20
  Bottom 0.152: v12.7,49.6 12.7,24.6 14.4,22.9 v14.4,19.8
CPTXLED  (via drill 0.3)
  Top 0.152: v22.66,19.06 21.52,20.2 19.3,20.2 19.05,19.95 U4.14 | v22.69,17.39 29,11.08 R15.1
  Bottom 0.152: v22.66,19.06 22.66,17.42 v22.69,17.39
DM
  Top 0.152: X1.D- 22.64,4.74 22.98,5.08 22.98,6.71 J12.P$1 18.36,11.35 18.36,14.65 18.55,14.85 U4.4
DP  (via drill 0.3)
  Top 0.152: X1.D+ 23.29,7.79 J11.P$1 | v19.54,9.34 19.38,9.49 19.38,9.88 18.05,11.22 U4.3
  Bottom 0.152: v19.54,9.34 20.57,9.34 20.85,9.62 22.48,9.62 J11.P$1
GND  (via drill 0.3, 0.35, 0.45)  (1 unrouted)
  Top 0.152: U1.60 13.75,58.85 15.45,57.15 | 15.45,57.15 U1.P$1 15.45,57.05 | 15.45,57.05 v13.5,55.1 12.75,54.35 U1.14 10.05,54.35 9.88,54.53 8.33,54.53 C1.2 | 15.45,57.15 15.25,56.95 U1.24 15.25,48.75 C3.2 | 15.65,56.85 18.65,53.85 U1.34 20.75,53.85 21.17,53.43 21.17,53.02 21.3,52.89 21.71,52.89 21.8,52.8 C4.2 | 15.65,56.85 15.45,57.05 | 17.7,58.85 U1.44 21.15,58.85 21.43,58.57 22.97,58.57 C5.2 | 17.7,58.85 17.65,58.85 15.65,56.85 | 17.7,58.85 17.75,58.9 U1.52 17.75,62.55 17.93,62.73 17.93,63.88 17.3,64.5 C6.2 | U4.2 17.55,17.55 v17.9,17.9 | C12.2 22,13.8 C13.2 21.01,13.4 v20.91,13.5
  Top 0.254: U2.4 6.24,20.13 U2.TH | U2.15 7.24,19.63 U2.TH | U2.14 7.24,19.13 U2.TH
  Top 0.305: X1.GND 24.59,6.59 J13.P$1
  other vias: 14,63.5 15.5,57.1 13.5,59.1 17.5,55.1 17.5,59.1 18.64,92.45 6.05,91.8 18.7,17 23.7,65.5 23.4,45.5 29.7,87.35 4.3,14.2 7.4,19 7.4,19.8 6.6,19.8 6.6,19 8.4,37 8.4,35 8.4,33 8.4,31 6.6,19.8 4.9,21.1
  pour Bottom: -2.5,115.5 52.5,115.5 52.5,-3 -2.5,-3
  pour Top (rank 2): 4,38.5 4,19.5 10,19.5 10,38.5
N$1
  Top 0.152: J3.GRNN 36.89,88.5 R2.2
N$2
  Top 0.152: J3.YLWN 36.87,77 R3.2
N$3
  Top 0.152: J4.GRNN 36.89,70 R4.2
N$4
  Top 0.152: J4.YLWN 36.87,58.5 R5.2
N$5
  Top 0.152: J5.GRNN 36.89,51.5 R6.2
N$6
  Top 0.152: J5.YLWN 36.87,40 R7.2
N$7
  Top 0.152: J6.GRNN 36.89,33 R8.2
N$8
  Top 0.152: J6.YLWN 36.87,21.5 R9.2
N$9
  Top 0.152: J7.GRNN 39.4,16.4 37.5,14.5 R10.2
N$10
  Top 0.152: J7.YLWN 36.87,3 R11.2
N$13
  Top 0.152: U1.58 14.75,63.3 Y1.1
N$14
  Top 0.152: U1.59 14.25,62.3 14.03,62.52 13.71,62.52 13.57,62.66 13.57,62.98 Y1.3
N$15
  Top 0.152: D3.2 R1.2
N$17
  Top 0.152: D4.2 R16.2
N$19
  Top 0.152: R12.2 22.71,15.54 22.71,16.01 21.47,17.25 U4.9
N$20
  Top 0.305: U2.10 6.74,16.54 C7.1
N$21
  Top 0.152: D5.2 R17.2
N$34  (via drill 0.3)
  Top 0.152: U2.9 5.8,17.91 v5.6,17.7
  Bottom 0.152: v5.6,17.7 5.6,16.19 U$1.2
N$37
  Top 0.152: D1.2 R14.2
N$38
  Top 0.152: D2.2 R15.2
PDI_DATA  (via drill 0.3)
  Top 0.152: U1.56 15.7,61.65 15.7,62.37 15.8,62.47 15.8,67.48 16.08,67.76 16.08,68.24 15.74,68.58 14.82,68.58 v14.5,68.9 | v13.7,83.7 13.56,83.84 J2.1
  Bottom 0.152: v14.5,68.9 14.5,82.9 v13.7,83.7
RESET/PDI_CLK  (via drill 0.3)
  Top 0.152: v17.9,83.1 18.64,83.84 J2.5 16.69,88.7 7.55,88.7 S1.P$4 | v15.5,68 15.5,62.6 15.25,62.35 U1.57
  Bottom 0.152: v17.9,83.1 15.5,80.7 v15.5,68
STLCLK  (via drill 0.3)
  Top 0.152: U1.62 12.62,61.73 12.62,62.05 12.18,62.48 11.9,62.48 11.9,64.82 12.1,65.02 12.44,65.02 12.78,65.36 12.78,65.7 v13.28,66.2 | v13.28,76.3 13.28,76.8 23.25,86.77 24.09,86.77 24.67,87.35 R16.1
  Bottom 0.152: v13.28,66.2 13.01,66.48 13.01,76.02 v13.28,76.3
STLERR  (via drill 0.3)
  Top 0.152: R17.1 13.05,77 v12.7,77 | U1.63 12.12,61.73 12.12,62.05 11.98,62.18 11.67,62.18 11.6,62.25 11.6,65 v12.2,65.6
  Bottom 0.152: v12.7,77 12.7,66.1 v12.2,65.6
VSW
  Top 0.305: U2.12 7.74,17.02 7.74,16.66 C7.2
  pour Top (no thermals): 7.5,17.5 7.5,22 4.5,22 4.5,25.5 9.5,25.5 9.5,17.5
VUSB  (via drill 0.3, 0.45, 0.55, 0.65)
  Top 0.152: v22,5.5 X1.VBUS | U4.8 21.15,16.75 v21.5,16.4
  Top 0.305: X1.VBUS 21.99,2.69 21.8,2.5 19.6,2.5 17.9,0.8 v16.6,0.8 | U2.11 7.24,16.87 7.29,16.83 7.29,14.6 | 7.29,14.6 7.29,14.38 C8.2 1.3,8.4 v1.3,8.2 | U2.3 U2.2 7.24,22.14 v7.6,22.5 | 7.29,14.6 8.28,15.6 8.71,15.6 10.5,17.39 v10.5,19.4
  Top 1.016: J10.P$1 v9.5,74
  Bottom 0.152: v22,5.5 18.7,8.8 18.7,9.6 21.5,12.4 21.5,15.08 21.42,15.16 21.42,15.64 21.5,15.72 v21.5,16.4
  Bottom 0.305: v7.6,22.5 9.2,22.5 10.5,21.2 v10.5,19.4
  Bottom 1.016: v16.6,0.8 11.2,0.8 4.5,7.5 2,7.5 v1.3,8.2 0.8,8.7 0.8,57.8 0.79,57.81 0.79,70.39 4.4,74 v9.5,74

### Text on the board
tPlace: err | clk | pwr | ATKP0 | reset | atkrouter v0.1 | ATKP1 | ATKP2 | ATKP3 | ATKP4 | rx atk | tx atk | tx bridge | rx bridge
bPlace: time is infinite / days go on forever / moments are lost / debugging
